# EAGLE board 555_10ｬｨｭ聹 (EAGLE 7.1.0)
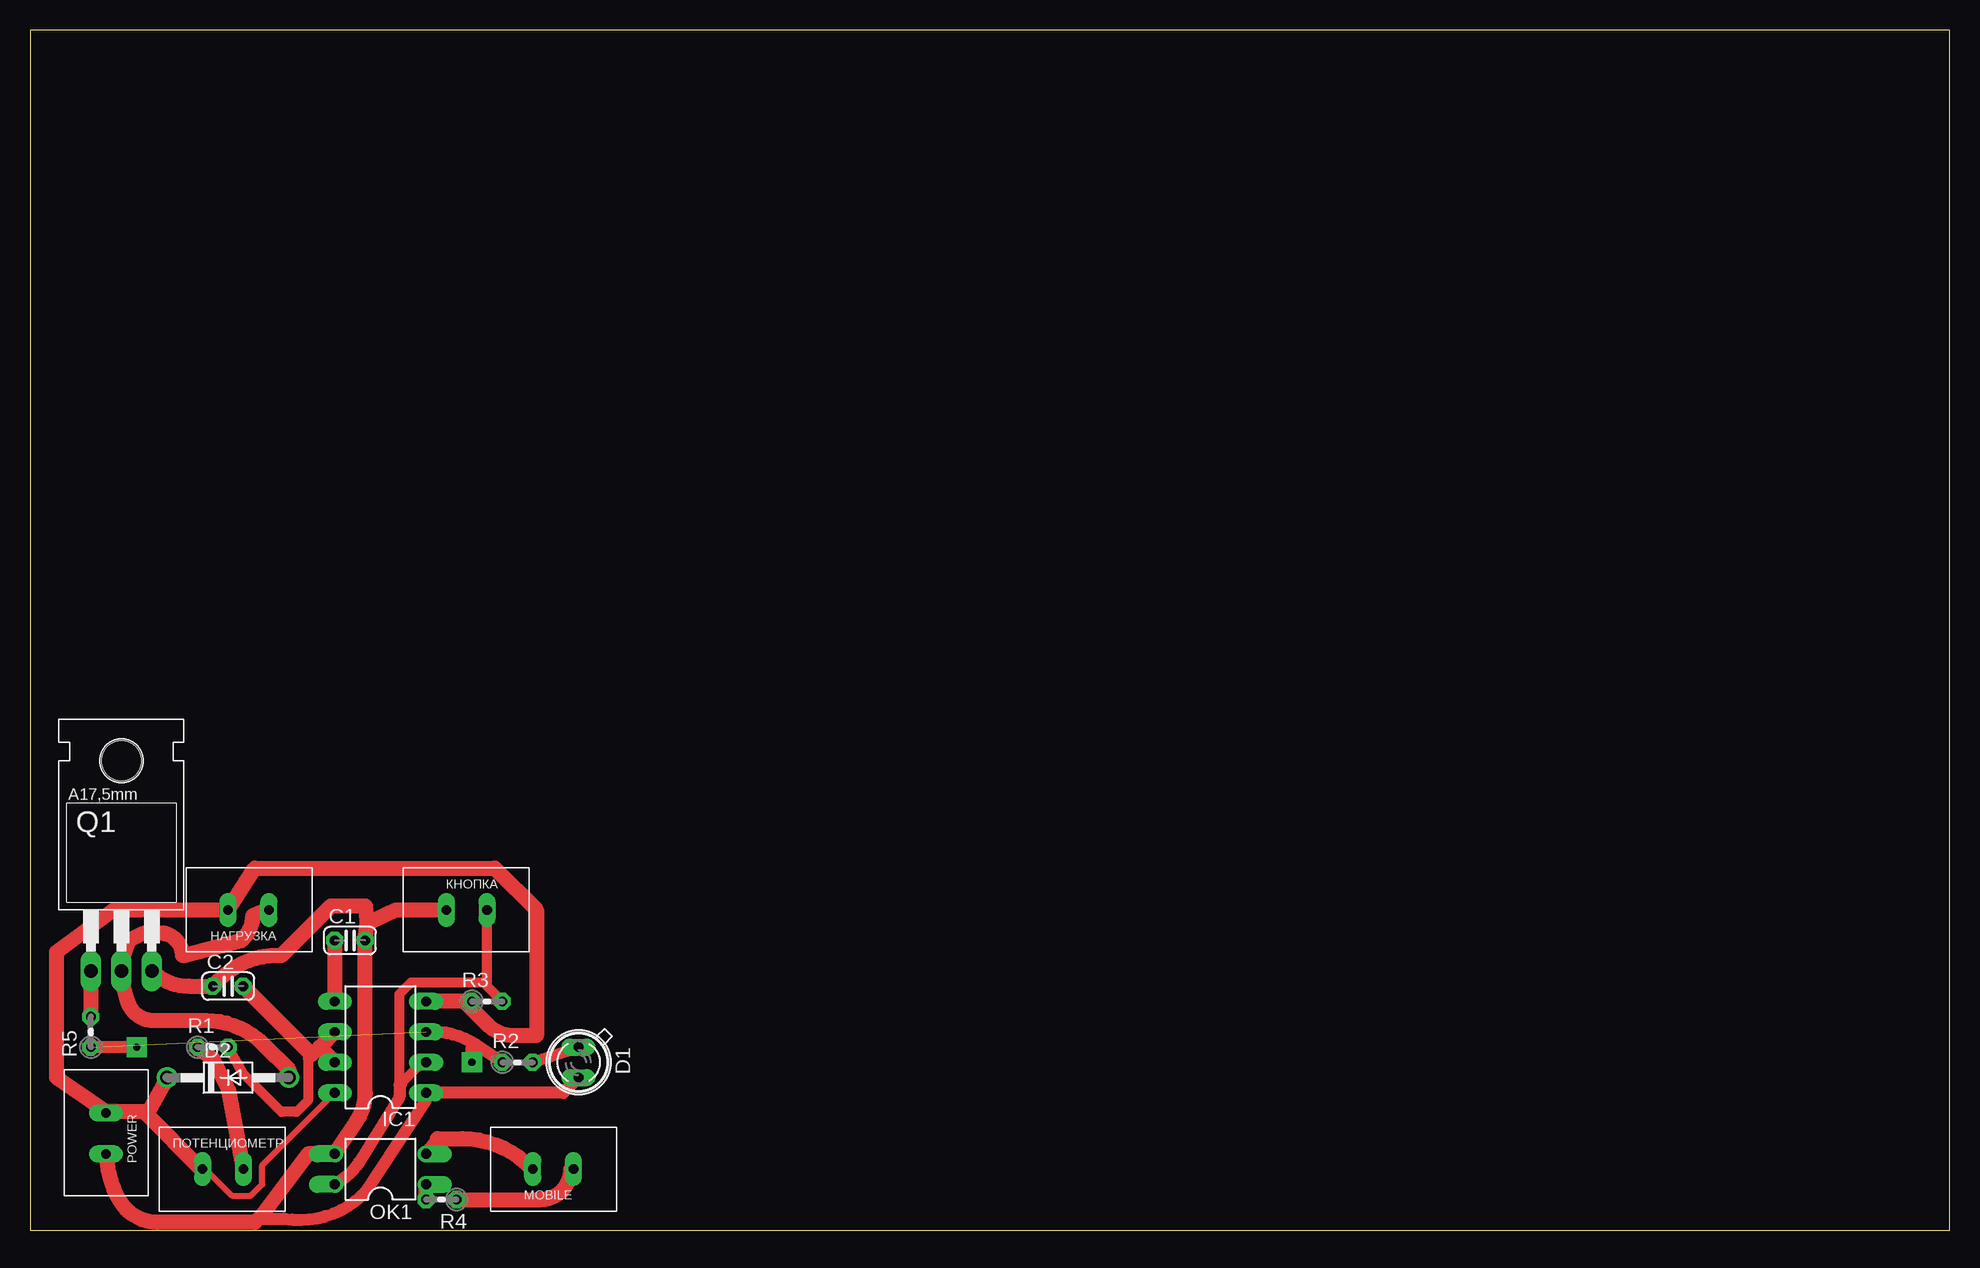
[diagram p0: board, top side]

Size 160 x 100 mm. Coordinates in mm from the lower left corner, seen from the top.
Outline: 0,0 160,0 160,100 0,100 0,0
Copper layers (1*16): Top 0.035mm / dielectric 1.5mm / Bottom 0.035mm
Design rules "default": minimum track width 20mil, minimum drill 32mil, track to track 14mil, track to pad 14mil, pad to pad 14mil, via to via 14mil, smd to smd 8mil, copper to edge 40mil, drill to drill 40mil, minimum pad ring 12mil, minimum via ring 12mil, stop-mask expansion 4mil, vias tented up to drill 0mil, thermal gap 10mil

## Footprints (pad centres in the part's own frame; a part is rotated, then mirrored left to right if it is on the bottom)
C025-024X044 = drill 0.813 octagon: 1 -1.27,0; 2 1.27,0
SFH482 = drill 0.813 long: A -1.27,0; K 1.27,0
DO41-10 = drill 1.118: A 5.08,0; C -5.08,0
DIL-08 = drill 0.813 long: 1 -3.81,-3.81; 2 -1.27,-3.81; 3 1.27,-3.81; 4 3.81,-3.81; 5 3.81,3.81; 6 1.27,3.81; 7 -1.27,3.81; 8 -3.81,3.81
CON2X3.4 = drill 0.8 long: P$1 0,0; P$2 3.4,0
DIL04 = drill 0.813 offset: 1 -1.27,-3.81; 2 1.27,-3.81; 3 1.27,3.81; 4 -1.27,3.81
TO220 = drill 1.118 long: 1 -2.54,-6.35; 2 0,-6.35; 3 2.54,-6.35 | hole 3.302: 0,11.176
0204V = drill 0.813 octagon: 1 -1.27,0; 2 1.27,0

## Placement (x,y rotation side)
C1  0.1mF  [C025-024X044]  26.67,24.13 0 top
C2  150mF  [C025-024X044]  16.51,20.32 0 top
D1  SFH482  [SFH482]  45.72,13.97 270 top
D2  1N4004  [DO41-10]  16.51,12.7 0 top
IC1  NE555  [DIL-08]  29.21,15.24 90 top
MOBILE  Вход звонка  [CON2X3.4]  41.91,5.08 0 top
OK1  PC817  [DIL04]  29.21,5.08 90 top
POWER  CON2X3.4  [CON2X3.4]  6.35,6.35 90 top
Q1  IRF540  [TO220]  7.62,27.94 0 top
R1  2.2m  [0204V]  15.24,15.24 0 top
R2  560  [0204V]  40.64,13.97 0 top
R3  10k  [0204V]  38.1,19.05 0 top
R4  1kOm  [0204V]  34.29,2.54 180 top
R5  560  [0204V]  5.08,16.51 90 top
КНОПКА  CON2X3.4  [CON2X3.4]  38.1,26.67 180 top
НАГРУЗКА  CON2X3.4  [CON2X3.4]  16.51,26.67 0 top
ПОТЕНЦИОМЕТР  CON2X3.4  [CON2X3.4]  17.78,5.08 180 top

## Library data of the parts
C1 C2 = resistor; SPICEPREFIX: C
D1 = led
D2 = diode
IC1 = st-microelectronics; MF: Arrow Electronics; MPN: NE555N; OC_FARNELL: 1467742; OC_NEWARK: 89K1486
MOBILE КНОПКА НАГРУЗКА ПОТЕНЦИОМЕТР = my
OK1 = optocoupler; MPN: PC817X4J000F; OC_FARNELL: 9707727; OC_NEWARK: 97K7059
POWER = my; QWE: 234
Q1 = transistor-fet
R1-R5 = resistor; SPICEPREFIX: R

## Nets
+12V: D2.C IC1.4 IC1.8 POWER.P$2 R3.1 НАГРУЗКА.P$1 ПОТЕНЦИОМЕТР.P$2
GND: C1.2 C2.1 D1.K IC1.1 OK1.3 POWER.P$1 Q1.3 КНОПКА.P$2
N$1: C2.2 IC1.6 IC1.7 R1.2
N$2: R1.1 ПОТЕНЦИОМЕТР.P$1
N$3: MOBILE.P$2 R4.1
N$4: IC1.3 R2.1 R5.1
N$5: D1.A R2.2
N$6: IC1.2 OK1.4 R3.2 КНОПКА.P$1
N$7: C1.1 IC1.5
N$8: OK1.1 R4.2
N$9: MOBILE.P$1 OK1.2
N$11: Q1.1 R5.2
N$12: D2.A Q1.2 НАГРУЗКА.P$2

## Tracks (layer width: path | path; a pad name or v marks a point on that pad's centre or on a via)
+12V
  Top 0.508: 9.84,9.84 9.53,9.84 | 14.29,5.08 ПОТЕНЦИОМЕТР.P$2 14.61,5.08 16.83,2.86 18.41,2.86 19.37,3.81 19.37,5.4 IC1.8 | 6.35,9.84 POWER.P$2
  Top 1.27: R3.1 36.2,19.05 | 36.2,19.05 IC1.4 | D2.C 9.84,9.84 | 14.29,5.08 9.53,9.84 6.35,9.84 2.22,12.7 2.22,23.18 6.99,26.67 НАГРУЗКА.P$1 18.73,30.16 38.73,30.16 42.23,26.67 42.23,16.19 40.41,16.19 arc-45 38.09,17.15 36.2,19.05
GND
  Top 0.508: 33.02,10.79 IC1.1 | 19.37,0.95 19.21,1.11
  Top 1.016: IC1.1 44.45,11.43 D1.K | 19.37,0.95 21.18,0.95 arc58 28.12,3.36 33.02,10.79
  Top 1.27: Q1.3 arc45 13.23,20.32 C2.1 15.78,20.86 arc-45 20.61,22.86 20.95,22.86 25.08,26.99 27.94,26.99 28.1,25.56 | КНОПКА.P$2 30.48,26.67 28.1,25.56 | 28.1,25.56 C1.2 27.94,11.38 arc-34 27.27,9.15 OK1.3 23.18,6.35 19.21,1.11 18.73,0.64 10.64,0.64 arc-59 7.51,2.41 arc-24 6.46,5.43 POWER.P$1
N$1
  Top 0.508: 24.13,15.24 23.5,14.61
  Top 0.813: R1.2 17.78,13.02 20.95,9.84 22.23,9.84 23.18,10.79 23.18,14.29 23.5,14.61
  Top 1.27: IC1.6 24.13,15.24 IC1.7 | 23.5,14.61 C2.2
N$2
  Top 1.27: ПОТЕНЦИОМЕТР.P$1 16.51,11.75 15.24,14.29 R1.1
N$3
  Top 0.508: 45.09,5.08 MOBILE.P$2
  Top 1.27: R4.1 42.55,2.54 arc90 45.09,5.08
N$4  (via drill 0.6 pad 1.68)  (1 unrouted)
  Top 1.016: R2.1 37.19,15.42 arc34 33.6,16.51 IC1.3 | v8.89,15.24 R5.1
N$5
  Top 1.016: R2.2 D1.A
N$6
  Top 0.508: 38.1,20.32 38.1,20.64 | IC1.2 32.7,13.97 | 30.8,12.38 30.96,12.22
  Top 0.813: КНОПКА.P$1 38.1,20.64 31.75,20.64 30.8,19.68 30.8,12.38 | R3.2 38.1,20.32 | 32.7,13.97 30.96,12.22
  Top 1.016: 30.96,12.22 30.8,12.06 30.8,11.11 27.42,5.65 arc-32 OK1.4
N$7
  Top 1.27: C1.1 IC1.5
N$8
  Top 1.27: R4.2 OK1.1
N$9
  Top 1.016: OK1.2 33.97,7.62
  Top 1.27: 33.97,7.62 36.03,7.62 arc-42 41.31,5.62 MOBILE.P$1
N$11
  Top 1.27: Q1.1 R5.2
N$12
  Top 0.508: Q1.2 7.62,22.23 | 19.68,26.67 НАГРУЗКА.P$2
  Top 1.27: 19.68,26.67 18.6,26.22 arc-45 17.63,24.13 12.7,22.86 arc90 10.79,24.77 9.53,24.77 8.26,24.13 7.62,22.23 | D2.A 21.59,13.34 19.43,15.49 arc45 14.67,17.46 10.29,17.46 arc-75 8.12,19.12 7.62,20.95 Q1.2
S$1  (via drill 0.6 pad 1.68)
  Top 1.016: v36.83,13.97 36.83,15.24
